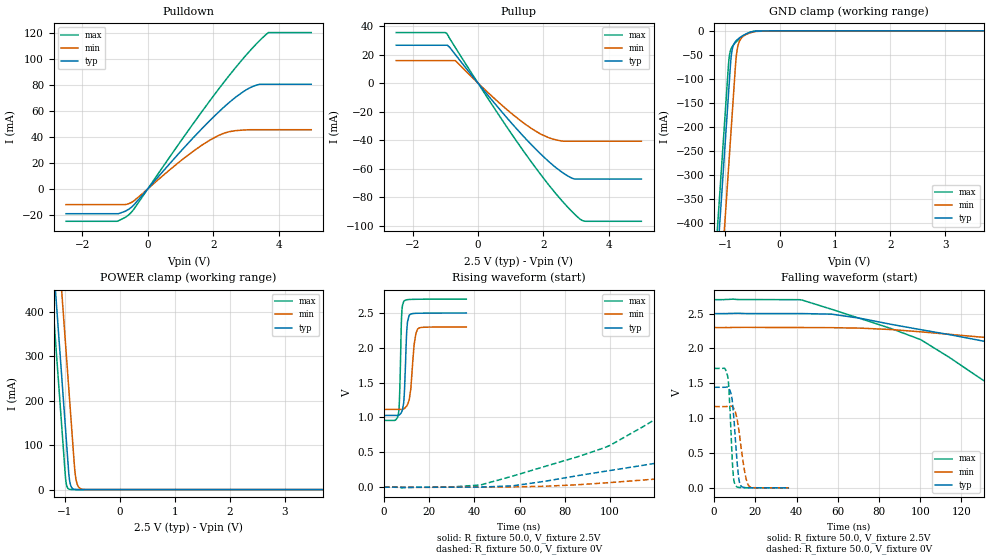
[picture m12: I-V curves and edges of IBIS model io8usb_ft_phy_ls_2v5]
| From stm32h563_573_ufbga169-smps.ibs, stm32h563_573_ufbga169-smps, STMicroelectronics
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[Model]   io8usb_ft_phy_ls_2v5
Model_type I/O
Polarity   Non-Inverting
Enable   Active-Low
| CAP_THRESHOLD on pad DPFT is "UDTCAPC" :
| Rising=20.0% of vddiom   Falling=80.0% of vddiom
| C_comp min and max val. don't necessarily correlate with the min and max pvt
| but are the smallest and greatest pad capacitance found.
| var   typ   min   max
C_comp   8.62848pF  8.50641pF  8.74957pF
|C_comp_pullup   5.79535pF  5.43180pF  5.42470pF
|C_comp_pulldown   2.83313pF  3.07461pF  3.32487pF
Vinl = 1.15V
Vinh = 1.35V
Vmeas = 1.25V   | Reference voltage for timing measurements
Cref  = 50.0pF   | Timing specification test load capacitance value
Rref  = 1.0MOhm   | Timing specification test load resistance value
Vref  = 1.375V   | Timing specification test load voltage
[Model Spec]
| TIME_THRESHOLD on pin ZIUSBPV11 is "CMOS" :
| Rising=40.0% of vdd   Falling=60.0% of vdd
Vinl 1.00380V 930.80000mV 1.08080V
Vinh 1.41920V 1.31220V 1.50720V
| variable   typ   min   max
[Temperature Range] 25.0 125.0 -40.0
| variable   typ   min   max
[Voltage Range] 2.5V 2.3V 2.7V
| variable   typ   min   max
[POWER Clamp Reference] 2.5V 2.3V 2.7V
| variable   typ   min   max
[GND Clamp Reference] 0V 0V 0V
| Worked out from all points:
|   slope of the pulldown table from 0 to 0.375 V, typ, clamps not added: 34.4 ohm
|   slope of the pullup table from 0 to 0.375 V, typ, clamps not added: 35.7 ohm
|   GND clamp passes 1 mA (typ) near -0.46 V on its own axis
|   POWER clamp passes 1 mA (typ) near -0.84 V on its own axis
|   rising waveform, R_fixture 50.0, V_fixture 2.5V: 20-80 % time 1.05ns typ, 1.81ns min, 780ps max; typ from 1.03 V to 2.5 V
|   falling waveform, R_fixture 50.0, V_fixture 2.5V: 20-80 % time 105ns typ, 188ns min, 66.3ns max; typ from 2.5 V to 1.03 V
|   rising waveform, R_fixture 50.0, V_fixture 0V: 20-80 % time 108ns typ, 199ns min, 67.1ns max; typ from 0 V to 1.44 V
|   falling waveform, R_fixture 50.0, V_fixture 0V: 20-80 % time 2.28ns typ, 3.38ns min, 1.66ns max; typ from 1.44 V to 0.001 V
[POWER Clamp]
-2.5V     2.708A     2.899A     2.597A
-1.29V    650.8mA    842.2mA    539.5mA
-1.2V     497.8mA    689.2mA    386.5mA
-1.18V    463.8mA    655.2mA    352.5mA
-1.12V    361.8mA    553.2mA    250.5mA
-1.05V    242.8mA    434.2mA    131.5mA
-980mV    123.8mA    315.2mA    17.95mA
-920mV    26.3mA     213.2mA    906uA
-810mV    363.5uA    33.6mA     3.797uA
-770mV    76.62uA    10.47mA    519.1nA
-700mV    5.028uA    1.361mA    16.38nA
5V        0A         0A         0A
[GND Clamp]
-2.5V     -2.787A    -2.944A    -2.726A
-1.21V    -594.3mA   -750.5mA   -532.8mA
-950mV    -152.3mA   -308.5mA   -90.81mA
-920mV    -101.3mA   -257.5mA   -50.71mA
-890mV    -54.53mA   -206.5mA   -37.29mA
-870mV    -38.94mA   -172.5mA   -32.93mA
-810mV    -22.25mA   -70.52mA   -24.51mA
-790mV    -19.71mA   -47.2mA    -22.19mA
-730mV    -14.01mA   -19.62mA   -15.92mA
-620mV    -6.579mA   -7.865mA   -6.951mA
-170mV    -138nA     -5.049uA   -5.744nA
5V        18.26nA    2.956uA    720.9pA
| variable   typ   min   max
[Pullup Reference] 2.5V 2.3V 2.7V
| variable   typ   min   max
[Pulldown Reference] 0V 0V 0V
[Pullup]
-2.5V     26.5mA     15.75mA    35.4mA
-960mV    26.5mA     15.75mA    35.01mA
-880mV    25.55mA    15.75mA    31.82mA
-690mV    19.93mA    15.75mA    24.85mA
870mV     -23.96mA   -18.3mA    -30.34mA
1.9V      -49.4mA    -35.58mA   -63.62mA
2.3V      -57.74mA   -39.37mA   -75.3mA
2.66V     -63.94mA   -40.84mA   -84.92mA
2.91V     -67.03mA   -40.84mA   -90.95mA
3.12V     -67.42mA   -40.84mA   -95.4mA
3.3V      -67.42mA   -40.84mA   -97.02mA
5V        -67.42mA   -40.84mA   -97.03mA
[Pulldown]
-2.5V     -19.1mA    -12.13mA   -24.93mA
-940mV    -19.1mA    -12.13mA   -24.93mA
-630mV    -16.37mA   -11.77mA   -20.86mA
-430mV    -12.46mA   -9.324mA   -15.74mA
960mV     27.48mA    20.57mA    34.9mA
1.9V      52.5mA     37.45mA    67.71mA
2.3V      62.12mA    42.45mA    80.97mA
2.7V      70.66mA    44.75mA    93.61mA
3.07V     76.91mA    45.37mA    104.5mA
3.4V      80.19mA    45.44mA    113.4mA
3.69V     80.36mA    45.44mA    120.1mA
5V        80.36mA    45.44mA    120.1mA
[Ramp]
dV/dt_r 866.07353mV/107.77491ns 700.02969mV/198.30257ns 1.02832V/66.89637ns
dV/dt_f 882.43539mV/104.11551ns 710.31132mV/187.90295ns 1.04513V/65.80405ns
R_load = 50.0
| Removed startup time: 0s 0s 0s  .
| Removed end time: 36.4ns.
[Rising Waveform]
R_fixture   = 50.0
V_fixture   = 2.5V
V_fixture_min = 2.3V
V_fixture_max = 2.7V
0s        1.029V     1.116V     958.1mV
6.55ns    1.033V     1.116V     1.085V
7ns       1.043V     1.115V     1.403V
7.8ns     1.078V     1.115V     2.45V
8.75ns    1.218V     1.123V     2.666V
10.1ns    2.251V     1.168V     2.689V
11.15ns   2.468V     1.25V      2.694V
13.4ns    2.494V     2.058V     2.696V
14.9ns    2.496V     2.269V     2.697V
36.4ns    2.499V     2.299V     2.699V
| Removed startup time: 0s 0s 0s  .
| Removed end time: 699.35ns.
[Falling Waveform]
R_fixture   = 50.0
V_fixture   = 2.5V
V_fixture_min = 2.3V
V_fixture_max = 2.7V
0s        2.5V       2.3V       2.7V
42.8ns    2.5V       2.3V       2.693V
100.3ns   2.269V     2.238V     2.124V
142.8ns   2.029V     2.13V      1.332V
190.2ns   1.575V     2.006V     1.013V
228.4ns   1.252V     1.894V     961.4mV
299.8ns   1.058V     1.597V     958.2mV
371.1ns   1.03V      1.307V     958.1mV
442.5ns   1.029V     1.178V     958.1mV
699.4ns   1.029V     1.116V     958.1mV
| Removed startup time: 0s 0s 0s  .
| Removed end time: 699.3ns.
[Rising Waveform]
R_fixture   = 50.0
V_fixture   = 0V
V_fixture_min = 0V
V_fixture_max = 0V
0s        15.7nV     1.095uV    10.18nV
42.8ns    774.6uV    684.2uV    32.24mV
97.4ns    226.2mV    60.08mV    565.2mV
142.7ns   476.4mV    171.5mV    1.369V
189.8ns   906mV      288.5mV    1.662V
228.4ns   1.222V     395.8mV    1.709V
299.7ns   1.419V     666.3mV    1.714V
371.1ns   1.442V     949.5mV    1.714V
442.5ns   1.443V     1.103V     1.714V
699.3ns   1.443V     1.167V     1.714V
| Removed startup time: 0s 0s 0s  .
| Removed end time: 36.35ns.
[Falling Waveform]
R_fixture   = 50.0
V_fixture   = 0V
V_fixture_min = 0V
V_fixture_max = 0V
0s        1.443V     1.167V     1.714V
6.6ns     1.446V     1.168V     1.6V
7.2ns     1.426V     1.171V     1.413V
9.15ns    1.152V     1.159V     244.2mV
10.4ns    667.8mV    1.082V     32.74mV
11.8ns    177.2mV    871.9mV    7.845mV
12.55ns   56.15mV    711.3mV    5.168mV
14.85ns   5.171mV    232.4mV    3.042mV
17.1ns    2.606mV    20.97mV    2.384mV
36.35ns   1.011mV    846.4uV    1.182mV
